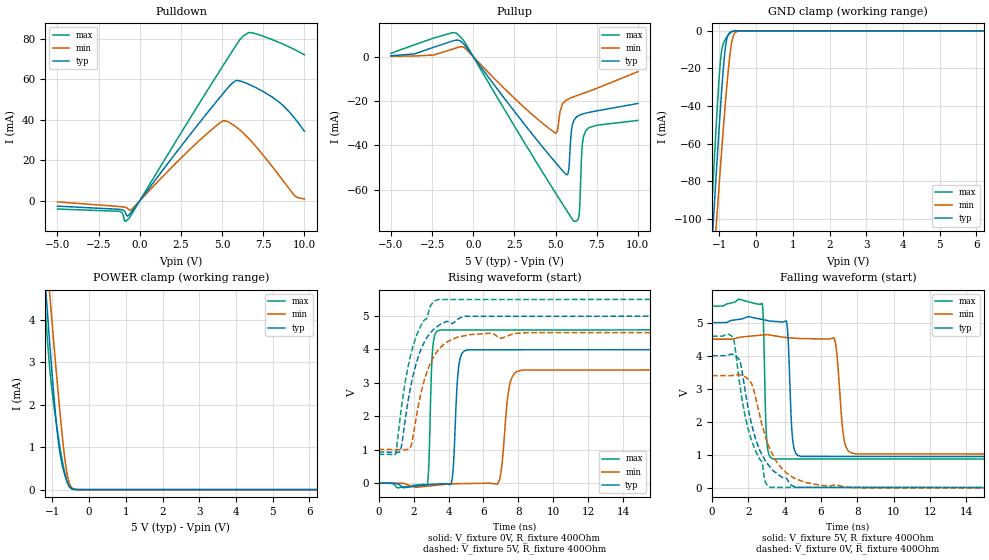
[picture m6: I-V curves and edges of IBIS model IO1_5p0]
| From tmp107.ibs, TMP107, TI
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|   Model
[Model]   IO1_5p0
Model_type   I/O
Polarity   Non-Inverting
Enable   Active-Low
Vinl = 1.5
Vinh = 3.5
Vmeas = 2.5
Vref = 0
Cref = 1pF
Rref = 100000
|   typ   min   max
C_comp   1.027pF   0.994pF   1.056pF
[Voltage Range]   5   4.5   5.5
[Temperature Range]   25   125   -55
[Pullup Reference]   5   4.5   5.5
[Pulldown Reference]   0   0   0
[Power Clamp Reference]   5   4.5   5.5
[GND Clamp Reference]   0   0   0
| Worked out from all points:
|   slope of the pulldown table from 0 to 0.75 V, typ, clamps not added: 91.8 ohm
|   slope of the pullup table from 0 to 0.75 V, typ, clamps not added: 99.8 ohm
|   GND clamp passes 1 mA (typ) near -0.72 V on its own axis
|   POWER clamp passes 1 mA (typ) near -0.82 V on its own axis
|   falling waveform, V_fixture 5V, R_fixture 400Ohm: 20-80 % time 180ps typ, 291ps min, 126ps max; typ from 5 V to 0.934 V
|   rising waveform, V_fixture 0V, R_fixture 400Ohm: 20-80 % time 219ps typ, 347ps min, 153ps max; typ from 0 V to 4 V
|   rising waveform, V_fixture 5V, R_fixture 400Ohm: 20-80 % time 1.11ns typ, 1.11ns min, 1.11ns max; typ from 0.934 V to 5 V
|   falling waveform, V_fixture 0V, R_fixture 400Ohm: 20-80 % time 1.21ns typ, 1.29ns min, 1.18ns max; typ from 4 V to 0 V
[Pulldown]
|   Voltage   I(typ)   I(min)   I(max)
-5V       -2.651mA   -561.2uA   -4.078mA
-1.25V    -4.213mA   -2.821mA   -5.186mA
-905mV    -5.349mA   -3.177mA   -10.08mA
-740mV    -7.563mA   -3.729mA   -9.371mA
-500mV    -5.463mA   -4.32mA    -6.749mA
3.16V     33.79mA    26.29mA    42.18mA
5.185V    54.24mA    39.59mA    68.45mA
5.83V     59.36mA    36.65mA    76.65mA
6.61V     57.65mA    30.9mA     83.19mA
8.56V     48.15mA    11.5mA     77.97mA
9.415V    40.74mA    2.449mA    74.73mA
10V       34.39mA    941.4uA    72.2mA
[GND Clamp]
|   Voltage   I(typ)   I(min)   I(max)
-5V       -1.45A     -1.264A    -1.625A
-1.25V    -129.6mA   -149.2mA   -110mA
-1.145V   -94.92mA   -119.7mA   -70.86mA
-1.07V    -70.86mA   -98.96mA   -44.49mA
-995mV    -47.81mA   -78.64mA   -21.66mA
-950mV    -34.83mA   -66.72mA   -12.19mA
-875mV    -15.98mA   -47.55mA   -5.982mA
-815mV    -5.94mA    -33.18mA   -3.817mA
-665mV    -367.9uA   -6.132mA   -589.3uA
-575mV    -61.56uA   -921.6uA   -83.46uA
-410mV    -1.079uA   -11.57uA   -577.1nA
10V       0A         0A         0A
[Pullup]
|   Voltage   I(typ)   I(min)   I(max)
-5V       414.5uA    192.9uA    1.528mA
-830mV    7.318mA    4.402mA    9.337mA
4.99V     -47.66mA   -34.36mA   -61.33mA
5.41V     -51.3mA    -21.46mA   -66.25mA
5.65V     -53.11mA   -19.6mA    -69.04mA
5.8V      -50.91mA   -18.98mA   -70.78mA
5.935V    -35.55mA   -18.54mA   -72.33mA
6.115V    -28.68mA   -18.01mA   -74.2mA
6.43V     -26.44mA   -17.17mA   -71.44mA
6.61V     -25.91mA   -16.7mA    -40.85mA
6.82V     -25.47mA   -16.14mA   -33.52mA
10V       -21.08mA   -6.74mA    -28.72mA
[POWER Clamp]
|   Voltage   I(typ)   I(min)   I(max)
-5V       53.72mA    48.48mA    61.69mA
-1.235V   5.364mA    6.322mA    4.791mA
-1.16V    4.464mA    5.522mA    3.823mA
-1.07V    3.415mA    4.573mA    2.832mA
-1.01V    2.743mA    3.949mA    2.329mA
-920mV    1.815mA    3.034mA    1.725mA
-800mV    893.7uA    1.873mA    1.03mA
-695mV    447uA      971.9uA    521.7uA
-620mV    232.1uA    468.4uA    244.8uA
-545mV    89.6uA     164.2uA    73.5uA
-470mV    22.47uA    43.79uA    12.2uA
10V       0A         0A         0A
[Ramp]
R_load = 400
|   typ   min   max
dV/dt_r   2.40012/2.17744e-10   2.03803/3.40883e-10   2.75453/1.53194e-10
dV/dt_f   2.43949/1.79061e-10   2.09445/2.89868e-10   2.78371/1.25332e-10
[Falling Waveform]
V_fixture = 5V
V_fixture_min = 4.5V
V_fixture_max = 5.5V
R_fixture = 400Ohm
C_fixture = 0F
|   Time   V(typ)   V(min)   V(max)
0s        5V         4.5V       5.5V
2.753ns   5.097V     4.625V     5.588V
3.01ns    5.068V     4.638V     1.444V
3.385ns   5.04V      4.607V     874.5mV
4.125ns   4.964V     4.549V     874.3mV
4.443ns   1.441V     4.535V     874.2mV
4.906ns   949.2mV    4.52V      874.1mV
6.728ns   948.6mV    4.522V     873.5mV
7.904ns   948.2mV    1.028V     873.2mV
50ns      934.2mV    1.009V     860.5mV
[Rising Waveform]
V_fixture = 0V
V_fixture_min = 0V
V_fixture_max = 0V
R_fixture = 400Ohm
C_fixture = 0F
|   Time   V(typ)   V(min)   V(max)
0s        127.1nV    178.7nV    101.2nV
2.773ns   -45.37mV   -90.8mV    -59.81mV
3.095ns   -31.84mV   -73.6mV    4.019V
3.495ns   -22.25mV   -52.22mV   4.577V
4.197ns   81.94mV    -20.22mV   4.577V
4.579ns   3.474V     -16.81mV   4.577V
5.096ns   3.985V     -12.22mV   4.577V
6.819ns   3.986V     -17.53mV   4.578V
8.21ns    3.986V     3.378V     4.578V
50ns      4V         3.397V     4.591V
[Rising Waveform]
V_fixture = 5V
V_fixture_min = 4.5V
V_fixture_max = 5.5V
R_fixture = 400Ohm
C_fixture = 0F
|   Time   V(typ)   V(min)   V(max)
0s        934.2mV    1.009V     860.5mV
963.8ps   920.1mV    1.004V     859.4mV
1.255ns   964.1mV    1.003V     2.046V
1.8ns     2.787V     1.046V     3.751V
2.153ns   3.587V     1.956V     4.386V
2.581ns   4.177V     3.012V     4.852V
3.385ns   4.69V      3.957V     5.488V
4.478ns   4.871V     4.357V     5.488V
6.433ns   4.987V     4.482V     5.489V
50ns      5V         4.5V       5.5V
[Falling Waveform]
|Gnd
V_fixture = 0V
V_fixture_min = 0V
V_fixture_max = 0V
R_fixture = 400Ohm
C_fixture = 0F
|   Time   V(typ)   V(min)   V(max)
0s        4V         3.397V     4.591V
1.184ns   4.028V     3.405V     4.497V
1.565ns   3.775V     3.418V     2.987V
1.972ns   2.457V     3.299V     1.813V
2.511ns   1.303V     2.466V     990.5mV
2.957ns   798.5mV    1.51V      144.5mV
3.248ns   593.4mV    1.094V     14.9mV
4.516ns   42.32mV    294.3mV    14.5mV
7.369ns   14.81mV    17.27mV    13.59mV
50ns      302nV      420nV      227.2nV
